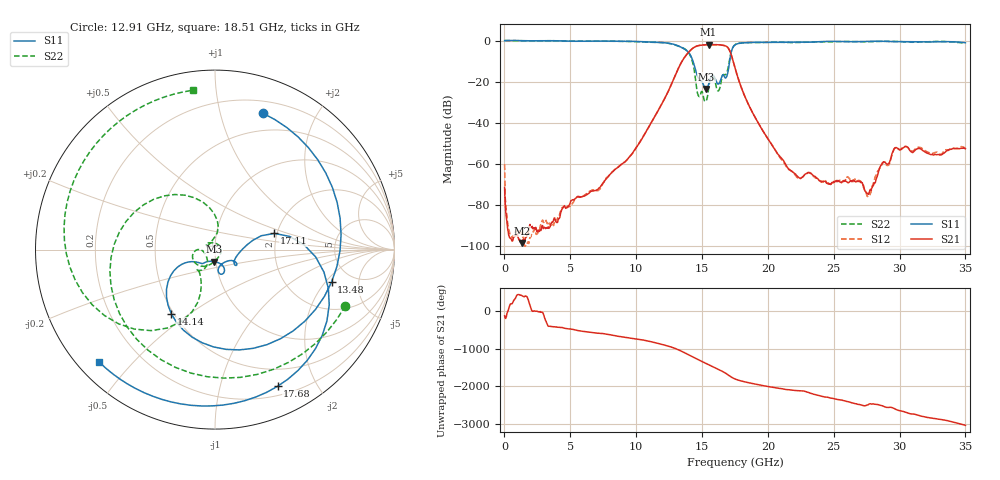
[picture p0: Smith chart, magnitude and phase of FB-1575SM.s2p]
! MARKI MICROWAVE INC.
! Email:  info@markimicrowave.com  Phone:  408-778-4200
! Model Number:  FB-1575SM  Date:  02/11
! Filename:		FB-1575SM.S2P  Version: 1.0
! Description:  2-port S-parameter data for Surface Mount Band Pass Filter FB-1575SM, measured in a connectorized fixture
! Frequency Range: 	10 MHz to 35 GHz
! Measurements:		S11, S21, S12, S22
# Hz S  dB  R 50
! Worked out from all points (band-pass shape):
!   801 points, 10 MHz to 35 GHz, reference 50 ohm
!   highest |S21| = -1.94 dB at 15.49 GHz (marker M1); lowest = -98.4 dB at 1.322 GHz (marker M2)
!   |S21| within 3 dB of the highest: 14.08 GHz to 17.1 GHz (3.024 GHz wide, 19.4 % of centre)
!   lowest |S11| = -23.5 dB at 15.32 GHz (marker M3), VSWR 1.14, Z = 48.9 - j6.55 ohm
!   |S11| at or under -10 dB: 14.31 GHz to 17.1 GHz (2.782 GHz wide, 17.7 % of centre)
!   |S22| runs from -29.6 to 0.1 dB; largest |S21 - S12| = 0.0012
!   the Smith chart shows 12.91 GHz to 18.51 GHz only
!   S11 on the Smith chart (normalised r, x): 12.91 GHz: 0.31, +1.36; 13.48 GHz: 3.51, -2.33; 14.14 GHz: 0.49, -0.43; 17.11 GHz: 1.93, +0.40; 17.68 GHz: 0.30, -1.52; 18.51 GHz: 0.06, -0.40
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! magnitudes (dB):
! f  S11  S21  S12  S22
! 10 MHz  0.0  -71.4  -60.2  0.1
! 272.4 MHz  0.1  -92.7  -90.3  0.1
! 1.322 GHz  0.0  -98.4  -94.7  0.0
! 5.871 GHz  -0.3  -76.1  -75.8  -0.2
! 9.501 GHz  -0.3  -56.4  -56.5  -0.3
! 11.69 GHz  -0.9  -33.8  -33.8  -0.8
! 12.91 GHz  -1.9  -17.7  -17.7  -2.0
! 13.48 GHz  -3.4  -10.0  -10.0  -3.3
! 14.14 GHz  -7.3  -4.6  -4.6  -7.7
! 14.71 GHz  -18.0  -2.5  -2.5  -26.5
! 15.32 GHz  -23.5  -2.0  -2.0  -29.3
! 15.49 GHz  -21.4  -1.9  -1.9  -23.6
! 17.11 GHz  -9.3  -5.0  -5.0  -8.6
! 17.5 GHz  -2.1  -13.2  -13.2  -2.0
! 17.68 GHz  -1.5  -17.0  -17.0  -1.4
! 18.51 GHz  -0.9  -30.8  -30.8  -1.0
! 21.53 GHz  -0.7  -62.0  -62.4  -0.9
! 23.37 GHz  -0.7  -65.2  -65.3  -0.7
! 27.65 GHz  -0.3  -74.7  -75.2  -0.5
! 29.18 GHz  -0.4  -59.8  -60.5  -0.3
! 29.75 GHz  -0.5  -52.0  -52.0  -0.4
! 35 GHz  -1.0  -52.6  -52.0  -1.2
